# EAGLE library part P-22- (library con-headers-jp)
HEADER PLUG PINS
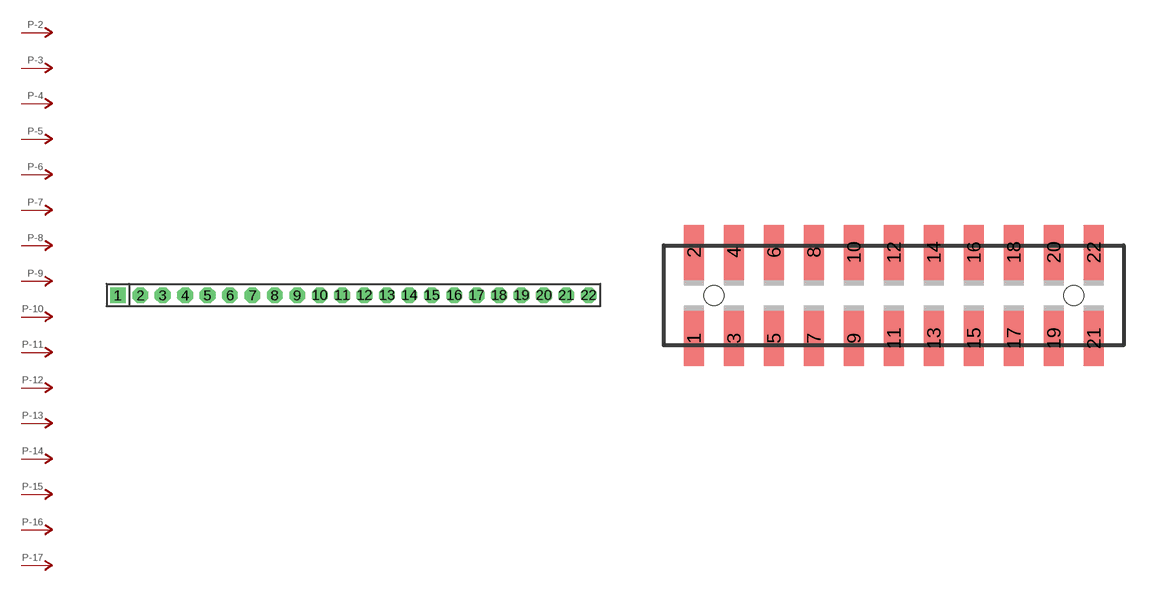
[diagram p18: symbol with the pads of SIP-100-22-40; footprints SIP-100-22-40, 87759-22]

Designator prefix P; gates -2=P-N -3=P-N -4=P-N -5=P-N -6=P-N -7=P-N -8=P-N -9=P-N -10=P-N -11=P-N -12=P-N -13=P-N -14=P-N -15=P-N -16=P-N -17=P-N -18=P-N -19=P-N -20=P-N -21=P-N -22=P-N -1=P-NV

## P-22-SIP-100-40  [SIP-100-22-40]
1  -1:P  pas
2  -2:P  pas
3  -3:P  pas
4  -4:P  pas
5  -5:P  pas
6  -6:P  pas
7  -7:P  pas
8  -8:P  pas
9  -9:P  pas
10  -10:P  pas
11  -11:P  pas
12  -12:P  pas
13  -13:P  pas
14  -14:P  pas
15  -15:P  pas
16  -16:P  pas
17  -17:P  pas
18  -18:P  pas
19  -19:P  pas
20  -20:P  pas
21  -21:P  pas
22  -22:P  pas

## P-22-87759  [87759-22]
Pads as for SIP-100-22-40

## P-22-100-2X11  [DIL-100-2X11]
Pads as for SIP-100-22-40

## P-22-100-2X11_M  [DIL-100-2X11_M]
Pads as for SIP-100-22-40

## P-22-2MM-2X11  [DIL-2MM-2X11]
Pads as for SIP-100-22-40

## P-22-2MM-2X11_M  [DIL-2MM-2X11_M]
Pads as for SIP-100-22-40

## P-22-SIP-100-32  [SIP-100-22-32]
Pads as for SIP-100-22-40

## P-22-SIP-100-40Y  [SIP-100-22-40Y]
Pads as for SIP-100-22-40

## P-22-SIP-100-32Y  [SIP-100-22-32Y]
Pads as for SIP-100-22-40

## P-22-87759_M  [87759-22_M]
Pads as for SIP-100-22-40

## Footprint SIP-100-22-40 (pad centres in mm)
SIP Header - 0.1", 40 mil drill
drill 1.016 pad 1.778 square: 1 -26.67,0
drill 1.016 pad 1.778 octagon: 2 -24.13,0; 3 -21.59,0; 4 -19.05,0; 5 -16.51,0; 6 -13.97,0; 7 -11.43,0; 8 -8.89,0; 9 -6.35,0; 10 -3.81,0; 11 -1.27,0; 12 1.27,0; 13 3.81,0; 14 6.35,0; 15 8.89,0; 16 11.43,0; 17 13.97,0; 18 16.51,0; 19 19.05,0; 20 21.59,0; 21 24.13,0; 22 26.67,0

## Footprint 87759-22 (pad centres in mm)
Molex PCB Pin Headers 2.00mm (.079") Pitch Milli-Grid Header, Vertical SMD
smd 1 x 2.75: 1 -10,-2.15; 2 -10,2.15; 3 -8,-2.15; 4 -8,2.15; 5 -6,-2.15; 6 -6,2.15; 7 -4,-2.15; 8 -4,2.15; 9 -2,-2.15; 10 -2,2.15; 11 0,-2.15; 12 0,2.15; 13 2,-2.15; 14 2,2.15; 15 4,-2.15; 16 4,2.15; 17 6,-2.15; 18 6,2.15; 19 8,-2.15; 20 8,2.15; 21 10,-2.15; 22 10,2.15
hole 1 at -9,0
hole 1 at 9,0

## Footprint DIL-100-2X11 (pad centres in mm)
PIN HEADER - 0.1"
drill 1.016 square: 1 -12.7,-1.27
drill 1.016 octagon: 2 -12.7,1.27; 3 -10.16,-1.27; 4 -10.16,1.27; 5 -7.62,-1.27; 6 -7.62,1.27; 7 -5.08,-1.27; 8 -5.08,1.27; 9 -2.54,-1.27; 10 -2.54,1.27; 11 0,-1.27; 12 0,1.27; 13 2.54,-1.27; 14 2.54,1.27; 15 5.08,-1.27; 16 5.08,1.27; 17 7.62,-1.27; 18 7.62,1.27; 19 10.16,-1.27; 20 10.16,1.27; 21 12.7,-1.27; 22 12.7,1.27

## Footprint DIL-100-2X11_M (pad centres in mm)
PIN HEADER - MIRRORED 0.1"
drill 1.016 square: 1 -12.7,1.27
drill 1.016 octagon: 2 -12.7,-1.27; 3 -10.16,1.27; 4 -10.16,-1.27; 5 -7.62,1.27; 6 -7.62,-1.27; 7 -5.08,1.27; 8 -5.08,-1.27; 9 -2.54,1.27; 10 -2.54,-1.27; 11 0,1.27; 12 0,-1.27; 13 2.54,1.27; 14 2.54,-1.27; 15 5.08,1.27; 16 5.08,-1.27; 17 7.62,1.27; 18 7.62,-1.27; 19 10.16,1.27; 20 10.16,-1.27; 21 12.7,1.27; 22 12.7,-1.27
